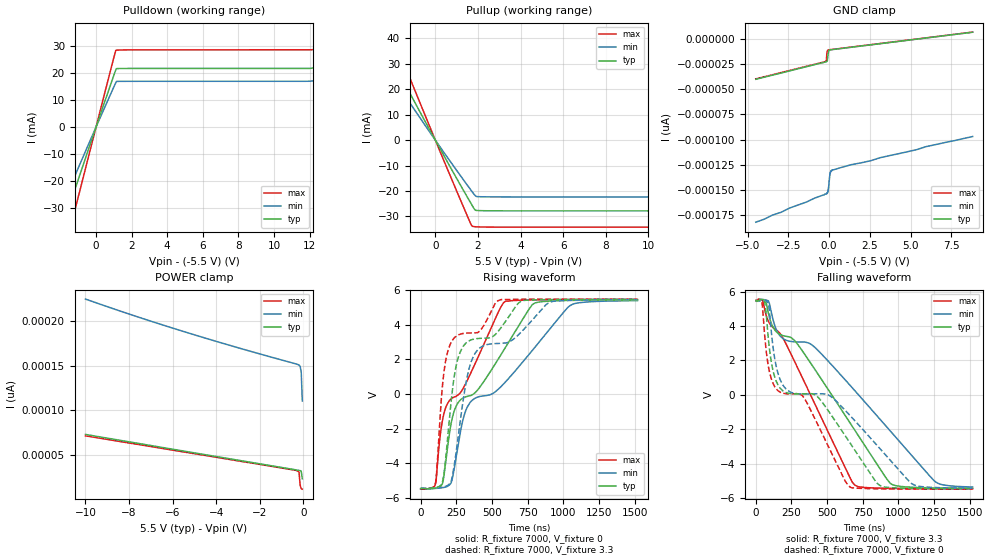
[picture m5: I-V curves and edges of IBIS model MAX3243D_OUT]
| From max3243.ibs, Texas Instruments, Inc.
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[Model]   MAX3243D_OUT
Model_type  3-state
Enable   Active-High
Vref =   0.0
Rref =   3000
Cref =   150p
Vmeas =   1.5
| variable   typ   min   max
C_comp   2.50pF   2.11pF   2.83pF
| C_pullup   2.74pF   2.10pF   3.19pF
| C_pulldown   2.74pF   2.10pF   3.19pF
| C_tri-state   2.50pF   2.11pF   2.83pF
[Temperature Range]   40   100   -40
| Ambient temperature   25   85   -40
|[Voltage range]   3.3   3   3.6
[GND Clamp Reference]   -5.5   -5.5   -5.5
[POWER Clamp Reference]   5.5   5.5   5.5
[Pulldown Reference]   -5.5   -5.5   -5.5
[Pullup Reference]   5.5   5.5   5.5
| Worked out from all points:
|   slope of the pulldown table from 0 to 1.65 V, typ, clamps not added: 75.8 ohm
|   slope of the pullup table from 0 to 1.65 V, typ, clamps not added: 67.2 ohm
|   rising waveform, R_fixture 7000, V_fixture 0: 20-80 % time 451ns typ, 597ns min, 339ns max; typ from -5.46 V to 5.43 V
|   falling waveform, R_fixture 7000, V_fixture 3.3: 20-80 % time 536ns typ, 873ns min, 381ns max; typ from 5.48 V to -5.41 V
|   rising waveform, R_fixture 7000, V_fixture 3.3: 20-80 % time 318ns typ, 416ns min, 121ns max; typ from -5.44 V to 5.47 V
|   falling waveform, R_fixture 7000, V_fixture 0: 20-80 % time 611ns typ, 771ns min, 462ns max; typ from 5.45 V to -5.45 V
[GND Clamp]
| MAX3243D_OUT_33
|   Voltage   I(typ)   I(min)   I(max)
-4.5V     -40.2pA    -182pA     -39.8pA
-265mV    -23.2pA    -154pA     -22.8pA
-175mV    -22.8pA    -154pA     -21.5pA
-150mV    -22.6pA    -154pA     -16.7pA
-110mV    -21.5pA    -153pA     -12.1pA
-65mV     -15.5pA    -151pA     -11.2pA
-20mV     -12.1pA    -145pA     -11pA
25mV      -11.3pA    -137pA     -10.9pA
60mV      -11.1pA    -133pA     -10.8pA
180mV     -10.8pA    -130pA     -10.6pA
5.95V     773fA      -107pA     940fA
8.8V      6.48pA     -97pA      6.63pA
[POWER Clamp]
| MAX3243D_OUT_33
|   Voltage   I(typ)   I(min)   I(max)
-10V      72.77pA    225.1pA    71.18pA
-7.85V    63.82pA    207.1pA    62.53pA
-5.5V     54.09pA    188.6pA    53.09pA
-3.1V     44.2pA     171.1pA    43.44pA
-400mV    33.13pA    152.5pA    32.59pA
-300mV    32.72pA    151.8pA    32.01pA
-200mV    32.3pA     150.9pA    30.3pA
-150mV    32.04pA    149.5pA    15.69pA
-100mV    31.47pA    143.1pA    11.66pA
-50mV     22.79pA    110.4pA    11.17pA
[Pulldown]
| MAX3243D_OUT_33
|   Voltage   I(typ)   I(min)   I(max)
-4.5V     -88.07mA   -69.2mA    -115.6mA
-2.57V    -50.42mA   -39.47mA   -66.52mA
-1.85V    -36.22mA   -28.3mA    -47.96mA
-1.545V   -30.21mA   -23.59mA   -40.08mA
-1.265V   -24.71mA   -19.27mA   -32.84mA
1.12V     21.39mA    16.6mA     28.54mA
12.18V    21.96mA    17.18mA    28.77mA
12.66V    23.84mA    18.62mA    31.23mA
13.26V    28.02mA    21.78mA    37.24mA
14.22V    37.63mA    29.03mA    51.03mA
15.09V    47.97mA    36.88mA    65.7mA
15.5V     53.38mA    41mA       73.31mA
[Pullup]
| MAX3243D_OUT_33
|   Voltage   I(typ)   I(min)   I(max)
-10V      147.7mA    116.6mA    197.5mA
-3.7V     57.5mA     45.68mA    75.82mA
-3.55V    55.17mA    43.83mA    72.76mA
-2.9V     45.07mA    35.78mA    59.47mA
-2.25V    34.93mA    27.71mA    46.12mA
-2V       31.03mA    24.61mA    40.98mA
550mV     -8.319mA   -6.582mA   -11.05mA
1.65V     -24.54mA   -19.39mA   -32.68mA
1.75V     -25.98mA   -20.53mA   -33.9mA
1.9V      -27.59mA   -22.03mA   -34.06mA
2.15V     -27.72mA   -22.25mA   -34.14mA
10V       -27.8mA    -22.32mA   -34.21mA
[Ramp]
| MAX3243D_OUT_33
| variable   typ   min   max
dV/dt_r   6.54/4.51E-07   6.51/5.97E-07   6.56/3.39E-07
dV/dt_f   6.58/5.47E-07   6.53/8.78E-07   6.60/3.86E-07
R_load = 7000
[Rising Waveform]
| MAX3243D_OUT_33
R_fixture =   7000
C_fixture =   0
L_fixture =   0
V_fixture =   0
V_fixture_min = 0
V_fixture_max = 0
|   Time   V(typ)   V(min)   V(max)
0s        -5.46V     -5.448V    -5.47V
103ns     -5.423V    -5.44V     -5.201V
152ns     -5.186V    -5.398V    -1.554V
208.5ns   -1.918V    -5.179V    -309.5mV
255.1ns   -589.3mV   -3.331V    -89.96mV
327.4ns   -128.7mV   -740.9mV   801.3mV
584.8ns   2.566V     618.7mV    5.298V
789.1ns   5.201V     2.583V     5.434V
1.05us    5.407V     5.121V     5.449V
1.52us    5.434V     5.396V     5.456V
[Falling Waveform]
| MAX3243D_OUT_33
R_fixture =   7000
C_fixture =   0
L_fixture =   0
V_fixture =   3.3
V_fixture_min = 3
V_fixture_max = 3.6
|   Time   V(typ)   V(min)   V(max)
0s        5.48V      5.471V     5.487V
48.42ns   5.527V     5.54V      5.459V
88.36ns   4.745V     5.456V     4.28V
179.2ns   3.476V     3.348V     3.46V
266ns     3.202V     3.086V     2.042V
392.1ns   1.755V     2.91V      -140.3mV
692.2ns   -2.021V    268.2mV    -5.21V
956.8ns   -5.199V    -2.222V    -5.422V
1.264us   -5.394V    -5.061V    -5.439V
1.52us    -5.414V    -5.346V    -5.444V
[Rising Waveform]
| MAX3243D_OUT_33
R_fixture =   7000
C_fixture =   0
L_fixture =   0
V_fixture =   3.3
V_fixture_min = 3
V_fixture_max = 3.6
|   Time   V(typ)   V(min)   V(max)
0s        -5.436V    -5.42V     -5.45V
106.3ns   -5.389V    -5.407V    -5.03V
150.7ns   -5.129V    -5.365V    281.2mV
240.8ns   1.289V     -3.808V    3.285V
329.5ns   3.026V     1.123V     3.525V
409.1ns   3.214V     2.63V      3.603V
563.9ns   3.834V     2.929V     5.453V
702.7ns   5.352V     3.564V     5.473V
915.5ns   5.458V     5.329V     5.48V
1.52us    5.474V     5.456V     5.484V
[Falling Waveform]
| MAX3243D_OUT_33
R_fixture =   7000
C_fixture =   0
L_fixture =   0
V_fixture =   0
V_fixture_min = 0
V_fixture_max = 0
|   Time   V(typ)   V(min)   V(max)
0s        5.449V     5.436V     5.461V
42.11ns   5.502V     5.506V     5.426V
88.28ns   3.254V     5.316V     1.666V
137.2ns   927.9mV    1.901V     419.8mV
199.7ns   188.5mV    460.4mV    84.28mV
336.6ns   66.81mV    57.07mV    -146.5mV
657.6ns   -2.747V    -1.166V    -5.322V
883.9ns   -5.31V     -3.239V    -5.449V
1.11us    -5.425V    -5.223V    -5.46V
1.52us    -5.447V    -5.416V    -5.466V
